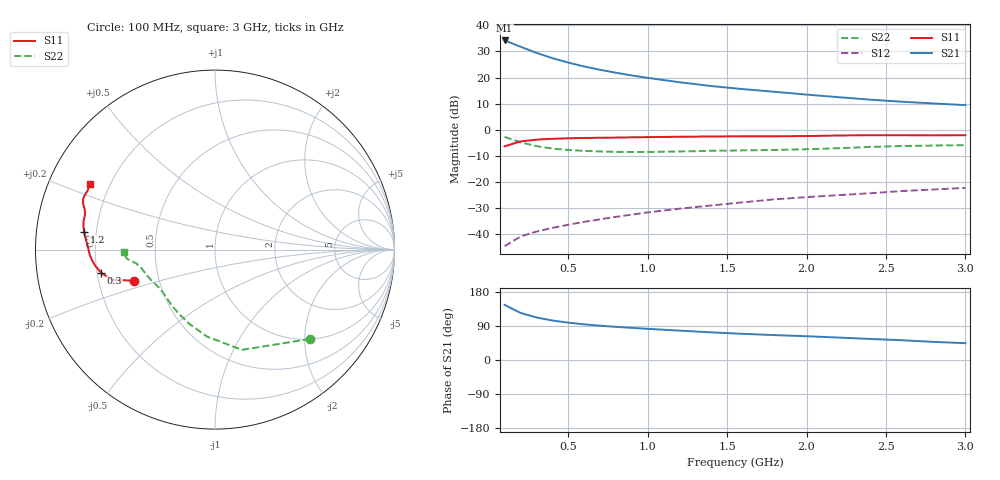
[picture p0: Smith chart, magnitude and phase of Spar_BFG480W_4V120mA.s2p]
! Filename: 4120BFG480.001
! Title: BFG480W
! Bias: Vce=4V; Ic=120mA
! Company: NXP Semiconductors NL
! User: Quality&Reliability T&D
! Measure time: 10 Nov 1999 / 12:04:25
#  MHz  S  MA  R 50
! Freq  S11  S21  S12  S22  :
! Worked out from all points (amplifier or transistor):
!   20 points, 100 MHz to 3 GHz, reference 50 ohm
!   highest |S21| = 34.2 dB at 100 MHz (marker M1)
!   |S21| within 3 dB of that: start of sweep to 226 MHz
!   unconditionally stable (mu >= 1): 640.6 MHz to end of sweep
!   at 400 MHz: K = 0.86, MSG = 32.5 dB, |S12| = -37.5 dB
!   at 1.2 GHz: K = 1.09, MAG = 22.4 dB, |S12| = -30.2 dB
!   at 3 GHz: K = 1.05, MAG = 14.5 dB, |S12| = -22.2 dB
!   S11 on the Smith chart (normalised r, x): 100 MHz: 0.36, -0.16; 300 MHz: 0.22, -0.10; 1.2 GHz: 0.15, +0.07; 3 GHz: 0.13, +0.24
100  0.4829 -159.0  51.2 145.4  0.00593 69.0  0.7269 -43.2
200  0.5982 -163.6  38.89 124.3  0.009076 60.9  0.5784 -75.0
300  0.6476 -168.5  29.66 112.2  0.01127 60.3  0.4862 -95.4
400  0.6727 -172.2  23.5 104.3  0.01327 62.7  0.4373 -109.3
500  0.6872 -175.0  19.33 98.6  0.01521 65.1  0.4107 -119.3
600  0.6978 -177.4  16.3 94.1  0.01731 67.0  0.395 -126.7
700  0.7035 -179.5  14.08 90.5  0.01934 69.2  0.3848 -132.4
800  0.7093 178.6  12.34 87.4  0.02156 70.8  0.3785 -137.1
900  0.7165 176.8  10.96 84.8  0.02379 72.4  0.376 -141.2
1000  0.7235 175.1  9.854 82.3  0.02628 73.4  0.3765 -144.9
1200  0.7356 172.2  8.128 77.5  0.03094 74.8  0.3849 -150.8
1400  0.7446 170.0  6.876 72.9  0.03562 75.6  0.3962 -155.1
1600  0.7495 167.7  5.996 69.0  0.04097 76.2  0.4034 -158.4
1800  0.7496 165.1  5.328 65.6  0.04673 76.6  0.4119 -162.0
2000  0.7589 162.9  4.716 62.7  0.05145 77.2  0.4241 -166.3
2200  0.7775 160.9  4.208 59.2  0.05607 76.9  0.4445 -169.9
2400  0.7874 159.1  3.77 55.6  0.06103 76.4  0.4694 -172.2
2600  0.7862 157.5  3.444 52.2  0.06728 75.6  0.4892 -173.6
2800  0.7823 155.2  3.192 47.8  0.072 74.2  0.4995 -175.4
3000  0.7872 152.5  2.964 44.4  0.07743 73.3  0.5077 -178.2
